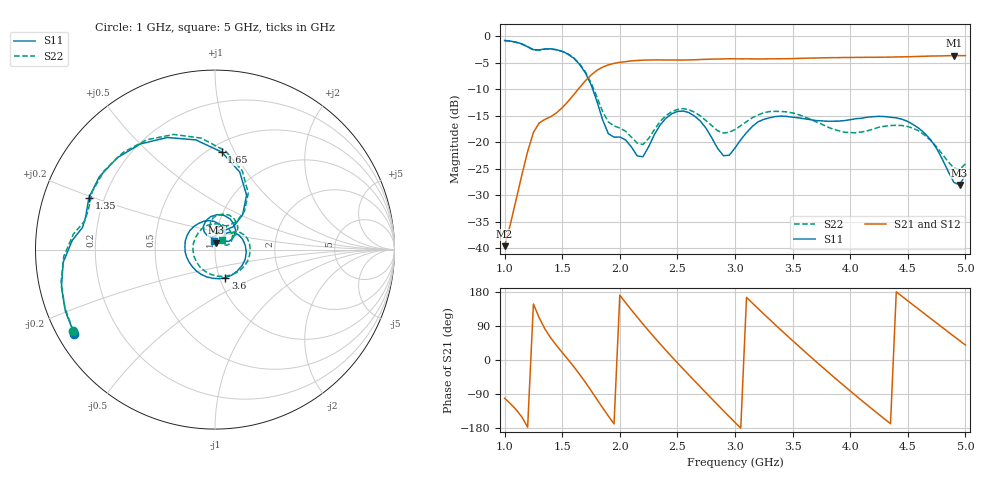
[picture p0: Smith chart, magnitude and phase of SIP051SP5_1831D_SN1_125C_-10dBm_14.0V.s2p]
# GHz  S  dB  R  50
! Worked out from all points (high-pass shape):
!   81 points, 1 GHz to 5 GHz, reference 50 ohm
!   highest |S21| = -3.64 dB at 4.9 GHz (marker M1); lowest = -39.6 dB at 1 GHz (marker M2)
!   |S21| within 3 dB of the highest: 1.789 GHz to end of sweep
!   lowest |S11| = -28.1 dB at 4.95 GHz (marker M3), VSWR 1.08, Z = 50.6 + j3.94 ohm
!   |S11| at or under -10 dB: 1.765 GHz to end of sweep
!   |S22| runs from -25.2 to -0.8 dB; largest |S21 - S12| = 0.0015
!   S11 on the Smith chart (normalised r, x): 1 GHz: 0.05, -0.28; 1.35 GHz: 0.14, +0.19; 1.65 GHz: 0.57, +0.89; 3.6 GHz: 1.07, -0.34; 5 GHz: 0.99, +0.10
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1  -0.79 -149.1  -39.62 -101.1  -39.61 -102.6  -0.81 -150.3
1.25  -2.52 170.4  -18.16 147.9  -18.17 147.5  -2.57 167.7
1.35  -2.39 157.7  -15.69 81.9  -15.67 81.8  -2.43 154.7
1.5  -2.84 125.2  -13.49 19.8  -13.48 19.8  -2.85 121.9
1.65  -5.27 86.1  -9.69 -37.3  -9.69 -37.1  -5.16 83.9
1.7  -6.87 72.3  -8.42 -58.4  -8.43 -58.2  -6.68 70.8
1.85  -15.71 51.3  -5.83 -125.6  -5.82 -125.6  -14.17 52.5
2  -19.00 79.2  -4.92 171.1  -4.90 171.2  -17.30 69.7
2.2  -22.75 105.6  -4.50 95.3  -4.50 95.4  -20.44 89.3
2.35  -16.73 116.5  -4.46 42.5  -4.45 42.6  -16.07 99.0
2.5  -14.19 86.4  -4.48 -7.4  -4.47 -7.4  -13.82 75.9
2.7  -16.01 43.5  -4.38 -71.3  -4.38 -71.3  -15.04 44.1
3  -21.08 57.3  -4.25 -164.7  -4.24 -164.7  -17.62 44.5
3.3  -15.38 8.0  -4.25 107.1  -4.26 107.0  -14.20 11.3
3.6  -15.56 -69.5  -4.15 23.7  -4.15 23.7  -15.17 -47.9
3.7  -15.90 -94.8  -4.10 -3.3  -4.10 -3.3  -16.12 -72.3
4  -15.75 -164.2  -4.00 -81.6  -4.00 -81.6  -18.19 -163.2
4.35  -15.28 122.0  -3.93 -168.1  -3.94 -168.1  -16.84 94.5
4.65  -18.38 63.6  -3.76 121.0  -3.77 120.9  -18.74 34.4
4.9  -27.58 57.9  -3.64 62.6  -3.65 62.6  -24.87 31.0
4.95  -28.06 79.5  -3.65 51.0  -3.65 51.0  -25.15 44.2
5  -26.11 95.3  -3.65 39.5  -3.64 39.4  -24.09 54.4
